FUNCTION_BLOCK FB_LN_IED_LD1_LEDGGIO8 EXTENDS FB_AcsiCommonLogicalNodeClass
VAR_INPUT
	NamPlt: FB_DO_IED_LD1_LEDGGIO8_NamPlt := (sClass:='LPL', bLinkResult:=THIS^.AddDataToContainer(ipData:=NamPlt));
	Beh: FB_DO_IED_LD1_LEDGGIO8_Beh := (sClass:='ENS', bLinkResult:=THIS^.AddDataToContainer(ipData:=Beh));
	Health: FB_DO_IED_LD1_LEDGGIO8_Health := (sClass:='ENS', bLinkResult:=THIS^.AddDataToContainer(ipData:=Health));
	Mod_: FB_DO_IED_LD1_LEDGGIO8_Mod := (sObjectName:='Mod', sClass:='ENC', bLinkResult:=THIS^.AddDataToContainer(ipData:=Mod_));
	AnOut1: FB_DO_IED_LD1_LEDGGIO8_AnOut1 := (sClass:='APC', bLinkResult:=THIS^.AddDataToContainer(ipData:=AnOut1));
	SPCSO1: FB_DO_IED_LD1_LEDGGIO8_SPCSO1 := (sClass:='SPC', bLinkResult:=THIS^.AddDataToContainer(ipData:=SPCSO1));
	DPCSO1: FB_DO_IED_LD1_LEDGGIO8_DPCSO1 := (sClass:='DPC', bLinkResult:=THIS^.AddDataToContainer(ipData:=DPCSO1));
	ISCSO1: FB_DO_IED_LD1_LEDGGIO8_ISCSO1 := (sClass:='INC', bLinkResult:=THIS^.AddDataToContainer(ipData:=ISCSO1));
END_VAR
VAR
END_VAR

END_FUNCTION_BLOCK
